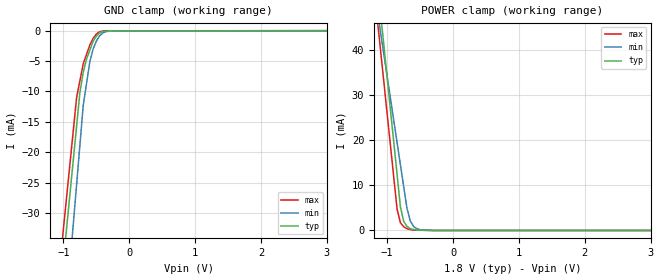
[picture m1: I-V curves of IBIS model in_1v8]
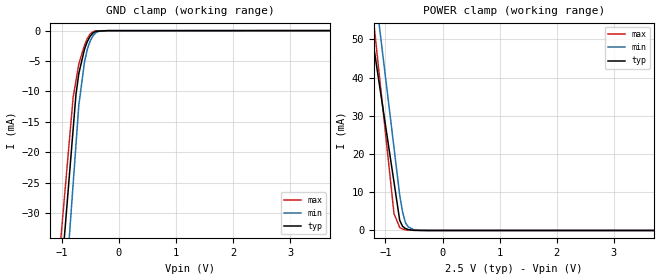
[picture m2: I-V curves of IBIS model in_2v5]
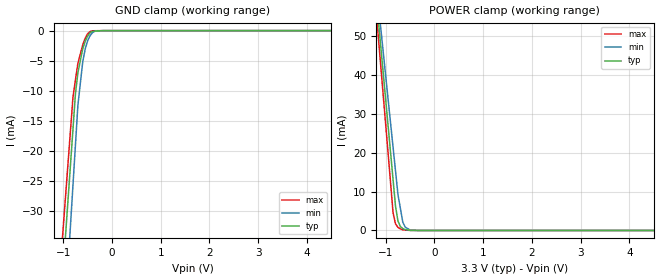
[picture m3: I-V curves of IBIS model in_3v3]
[IBIS Ver]   3.2
[Comment Char] |_char
[File Name]   ads1278_sp.ibs
[File Rev]   3.0
[Source]
| This model file was created by Teraspeed Consulting Group LLC
| (http://www.teraspeed.com/).
[Date]   01-14-2008
[Notes]   Quality Check of this IBIS model: Model Passes IBIS Check
   Model parses into ICX IS. Simulation done with Hyperlynx.
   1. MIN TYP MAX information is based on Temprature and Voltage
   characteristics only.
[Disclaimer]
| This model is designed as an aid for customers of Texas Instruments.
| TI and its licensors and suppliers make no warranties, either expressed
| or implied, with respect to this  model, including the warranties of
| merchantability or fitness for a particular purpose.
| The model is provided solely on an "as is" basis. The entire risk as to
| its quality and performance is with the customer.
[Copyright]
| (C) Copyright 2008 Texas Instruments Incorporated. All rights reserved.
[Component]   ADS1278-SP
[Manufacturer] TI
[Package]
| variable   typ   min   max
R_pkg  6.05E-02  5.80E-02  6.50E-02
L_pkg  5.05E-09  4.85E-09  5.38E-09
C_pkg  2.68E-13  2.40E-13  3.00E-13
[Pin] signal_name  model_name  R_pin  L_pin C_pin
1   AINP2   analog   6.50E-02   5.38E-09   3.00E-13
2   AINN2   analog   6.30E-02   5.25E-09   2.90E-13
3   AINP1   analog   6.20E-02   5.13E-09   2.80E-13
4   AINN1   analog   6.00E-02   5.04E-09   2.70E-13
5   AVDD   POWER   5.90E-02   4.95E-09   2.60E-13
6   AGND   GND   5.90E-02   4.90E-09   2.50E-13
7   DGND   GND   5.80E-02   4.87E-09   2.50E-13
8   TEST0   input   5.80E-02   4.85E-09   2.40E-13
9   TEST1   input   5.80E-02   4.85E-09   2.40E-13
10   CLKDIV   input   5.80E-02   4.87E-09   2.50E-13
11   _SYNC   input   5.90E-02   4.90E-09   2.50E-13
12   DIN   input   5.90E-02   4.95E-09   2.60E-13
13   DOUT8   output   6.00E-02   5.04E-09   2.70E-13
14   DOUT7   output   6.20E-02   5.13E-09   2.80E-13
15   DOUT6   output   6.30E-02   5.25E-09   2.90E-13
16   DOUT5   output   6.50E-02   5.38E-09   3.00E-13
17   DOUT4   output   6.50E-02   5.38E-09   3.00E-13
18   DOUT3   output   6.30E-02   5.25E-09   2.90E-13
19   DOUT2   output   6.20E-02   5.13E-09   2.80E-13
20   DOUT1   output   6.00E-02   5.04E-09   2.70E-13
21   DGND   GND   5.90E-02   4.95E-09   2.60E-13
22   IOVDD   POWER   5.90E-02   4.90E-09   2.50E-13
23   IOVDD   POWER   5.80E-02   4.87E-09   2.50E-13
24   DGND   GND   5.80E-02   4.85E-09   2.40E-13
25   DGND   GND   5.80E-02   4.85E-09   2.40E-13
26   DVDD   POWER   5.80E-02   4.87E-09   2.50E-13
27   CLK   input   5.90E-02   4.90E-09   2.50E-13
28   SCLK   out_io   5.90E-02   4.95E-09   2.60E-13
29   _DRDY/FSYNC out_io   6.00E-02   5.04E-09   2.70E-13
30   FORMAT2   input   6.20E-02   5.13E-09   2.80E-13
31   FORMAT1   input   6.30E-02   5.25E-09   2.90E-13
32   FORMAT0   input   6.50E-02   5.38E-09   3.00E-13
33   MODE1   input   6.50E-02   5.38E-09   3.00E-13
34   MODE0   input   6.30E-02   5.25E-09   2.90E-13
35   _PWDN8   input   6.20E-02   5.13E-09   2.80E-13
36   _PWDN7   input   6.00E-02   5.04E-09   2.70E-13
37   _PWDN6   input   5.90E-02   4.95E-09   2.60E-13
38   _PWDN5   input   5.90E-02   4.90E-09   2.50E-13
39   _PWDN4   input   5.80E-02   4.87E-09   2.50E-13
40   _PWDN3   input   5.80E-02   4.85E-09   2.40E-13
41   _PWDN2   input   5.80E-02   4.85E-09   2.40E-13
42   _PWDN1   input   5.80E-02   4.87E-09   2.50E-13
43   AGND   GND   5.90E-02   4.90E-09   2.50E-13
44   AVDD   POWER   5.90E-02   4.95E-09   2.60E-13
45   AINP8   analog   6.00E-02   5.04E-09   2.70E-13
46   AINN8   analog   6.20E-02   5.13E-09   2.80E-13
47   AINP7   analog   6.30E-02   5.25E-09   2.90E-13
48   AINN7   analog   6.50E-02   5.38E-09   3.00E-13
49   AINP6   analog   6.50E-02   5.38E-09   3.00E-13
50   AINN6   analog   6.30E-02   5.25E-09   2.90E-13
51   AINP5   analog   6.20E-02   5.13E-09   2.80E-13
52   AINN5   analog   6.00E-02   5.04E-09   2.70E-13
53   AVDD   POWER   5.90E-02   4.95E-09   2.60E-13
54   AGND   GND   5.90E-02   4.90E-09   2.50E-13
55   VCOM   analog   5.80E-02   4.87E-09   2.50E-13
56   VREFP   analog   5.80E-02   4.85E-09   2.40E-13
57   VREFN   analog   5.80E-02   4.85E-09   2.40E-13
58   AGND   GND   5.80E-02   4.87E-09   2.50E-13
59   AGND   GND   5.90E-02   4.90E-09   2.50E-13
60   AVDD   POWER   5.90E-02   4.95E-09   2.60E-13
61   AINP4   analog   6.00E-02   5.04E-09   2.70E-13
62   AINN4   analog   6.20E-02   5.13E-09   2.80E-13
63   AINP3   analog   6.30E-02   5.25E-09   2.90E-13
64   AINN3   analog   6.50E-02   5.38E-09   3.00E-13
[Diff Pin] inv_pin vdiff tdelay_typ tdelay_min tdelay_max
1   2   NA  NA  NA  NA
3   4   NA  NA  NA  NA
45  46  NA  NA  NA  NA
47  48  NA  NA  NA  NA
49  50  NA  NA  NA  NA
51  52  NA  NA  NA  NA
56  57  NA  NA  NA  NA
61  62  NA  NA  NA  NA
63  64  NA  NA  NA  NA
[Model Selector]  input
in_1v8   1.8V digital input
in_2v5   2.5V digital input
in_3v3   3.3V digital input
[Model Selector]  output
out_1v8  1.8V digital output
out_2v5  2.5V digital output
out_3v3  3.3V digital output
[Model Selector]  out_io
io_1v8   1.8V digital io
io_2v5   2.5V digital io
io_3v3   3.3V digital io
[Model] analog
Model_type Terminator
C_comp   0  0  0
| variable   typ   min   max
[Voltage Range]   5.00000V  4.75000V  5.25000V
[POWER Clamp Reference]  5.00000V  4.75000V  5.25000V
[GND Clamp Reference]   0.00000V  0.00000V  0.00000V
[Temperature Range]   25   105   -40
| Models and submodels in the file (10): analog (Terminator), in_1v8 (Input), in_2v5 (Input), in_3v3 (Input), io_1v8 (I/O), io_2v5 (I/O), io_3v3 (I/O), out_1v8 (Output), out_2v5 (Output), out_3v3 (Output)
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[Model] in_1v8
Model_type Input
Vinl = 540.000mV
Vinh = 1.26000V
C_comp 550.00fF 550.00fF 550.00fF
| variable typ   min   max
[Voltage Range] 1.80000V 1.65000V 1.95000V
[POWER Clamp Reference] 1.80000V 1.65000V 1.95000V
[GND Clamp Reference] 0.00000V 0.00000V 0.00000V
[Temperature Range]   25   105   -40
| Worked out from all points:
|   GND clamp passes 1 mA (typ) near -0.51 V on its own axis
|   POWER clamp passes 1 mA (typ) near -0.71 V on its own axis
[GND Clamp]
-1.8V     -126.5mA   -155.1mA   -119.2mA
-800mV    -15.68mA   -25.31mA   -10.98mA
-750mV    -10.14mA   -18.82mA   -8.217mA
-700mV    -6.854mA   -12.33mA   -5.455mA
-650mV    -4.678mA   -8.736mA   -3.914mA
-600mV    -3.206mA   -5.142mA   -2.373mA
-550mV    -1.733mA   -3.037mA   -1.263mA
-500mV    -879.1uA   -1.691mA   -533.2uA
-450mV    -347.6uA   -835.1uA   -153.4uA
-350mV    -72.58uA   -111.4uA   -21.33uA
-175mV    -839nA     -26.7uA    -3.137uA
3.6V      11.89uA    31.95uA    7.393uA
[POWER Clamp]
-1.8V     147.3mA    111.6mA    137.7mA
-1V       33.7mA     34mA       25.71mA
-850mV    12.4mA     19.45mA    4.715mA
-800mV    5.3mA      14.6mA     1.738mA
-750mV    2.037mA    9.746mA    815.9uA
-700mV    878.6uA    4.895mA    411.1uA
-650mV    420.9uA    2.129mA    185.9uA
-600mV    208.4uA    889.4uA    64.99uA
-550mV    77.29uA    389.7uA    56.32uA
-500mV    63.24uA    166.4uA    47.66uA
-300mV    7.027uA    0A         13uA
3.6V      0A         0A         0A
[Model] in_2v5
Model_type Input
Vinl = 750.000mV
Vinh = 1.75000V
C_comp 550.00fF 550.00fF 550.00fF
| variable typ   min   max
[Voltage Range] 2.50000V 2.25000V 2.75000V
[POWER Clamp Reference] 2.50000V 2.25000V 2.75000V
[GND Clamp Reference] 0.00000V 0.00000V 0.00000V
[Temperature Range]   25   105   -40
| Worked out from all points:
|   GND clamp passes 1 mA (typ) near -0.51 V on its own axis
|   POWER clamp passes 1 mA (typ) near -0.69 V on its own axis
[GND Clamp]
-2.5V     -212.8mA   -246.6mA   -194.3mA
-800mV    -16.27mA   -25.27mA   -11.01mA
-750mV    -10.49mA   -18.76mA   -8.233mA
-700mV    -7.041mA   -12.25mA   -5.455mA
-600mV    -3.027mA   -5.106mA   -2.372mA
-550mV    -1.774mA   -3.015mA   -1.262mA
-500mV    -907.6uA   -1.677mA   -532.7uA
-450mV    -365.3uA   -827.1uA   -153.3uA
-400mV    -103.8uA   -338.8uA   -27.27uA
-350mV    -78.65uA   -109.9uA   -20.53uA
-175mV    -3.148uA   -6.451uA   -264.8nA
5V        5.271uA    10.52uA    7.001uA
[POWER Clamp]
-2.5V     177.3mA    226.1mA    236.9mA
-1.1V     37.56mA    52.6mA     39.62mA
-1.05V    32.57mA    46.41mA    32.58mA
-850mV    12.62mA    21.62mA    4.401mA
-750mV    2.64mA     9.23mA     778.1uA
-700mV    1.09mA     4.865mA    395.7uA
-650mV    507.8uA    2.059mA    175uA
-600mV    239uA      932.4uA    61.37uA
-500mV    29.92uA    179.1uA    46.93uA
-400mV    17.95uA    21.5uA     32.49uA
5V        0A         0A         0A
[Model] in_3v3
Model_type Input
Vinl = 990.000mV
Vinh = 2.31000V
C_comp 550.00fF 550.00fF 550.00fF
| variable typ   min   max
[Voltage Range] 3.30000V 3.00000V 3.60000V
[POWER Clamp Reference] 3.30000V 3.00000V 3.60000V
[GND Clamp Reference] 0.00000V 0.00000V 0.00000V
[Temperature Range]   25   105   -40
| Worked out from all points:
|   GND clamp passes 1 mA (typ) near -0.51 V on its own axis
|   POWER clamp passes 1 mA (typ) near -0.70 V on its own axis
[GND Clamp]
-3.3V     -306.8mA   -355.6mA   -282mA
-800mV    -16.32mA   -25.63mA   -11.01mA
-750mV    -10.51mA   -19.03mA   -8.231mA
-700mV    -7.039mA   -12.43mA   -5.452mA
-600mV    -3.025mA   -5.175mA   -2.372mA
-550mV    -1.771mA   -3.054mA   -1.262mA
-500mV    -905.9uA   -1.699mA   -533uA
-450mV    -364uA     -838.7uA   -153.3uA
-400mV    -103.5uA   -344.4uA   -27.19uA
-350mV    -78.42uA   -111.8uA   -20.48uA
-175mV    -3.132uA   -5.9uA     -327.7nA
6.6V      5.71uA     6.995uA    1.843uA
[POWER Clamp]
-3.3V     345.7mA    318.5mA    371.2mA
-1.15V    53.77mA    57.76mA    49.43mA
-1.1V     46.99mA    51.7mA     41.94mA
-1.05V    40.2mA     45.64mA    34.46mA
-850mV    13.05mA    21.39mA    4.525mA
-800mV    6.26mA     15.32mA    1.711mA
-750mV    2.428mA    9.261mA    801.4uA
-700mV    1.019mA    5.681mA    407.6uA
-650mV    482.3uA    2.1mA      184.6uA
-600mV    224.1uA    846uA      102.7uA
-450mV    21.24uA    66.34uA    15.88uA
6.6V      0A         0A         0A
